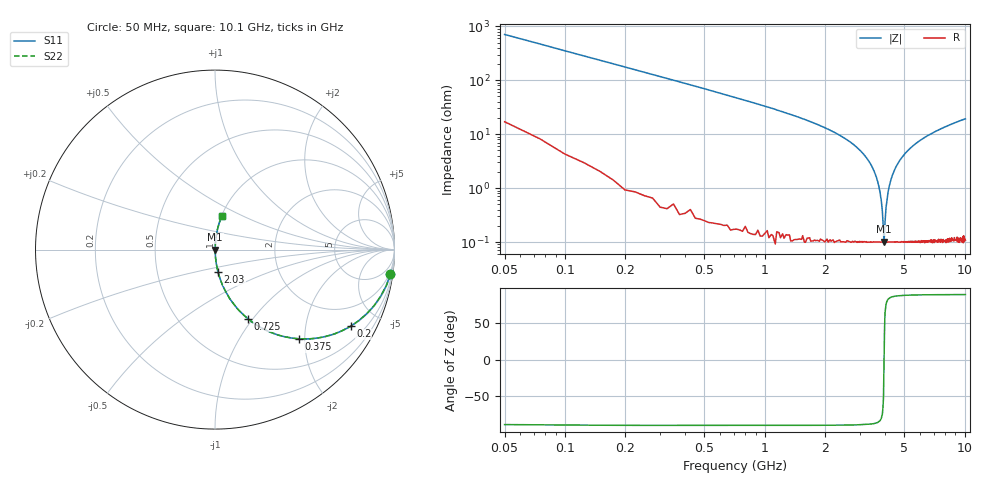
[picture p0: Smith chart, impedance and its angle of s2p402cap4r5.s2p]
! AVX Thin Film Operation		Date: April 2003
! Description: Accu-P® Series, Thin Film, SMD, RF Capacitor
! Part Number: 04025J4R5ABS
! 50 MHz  -  10.05 GHz
! Serial Measurements
# hz S db R 50
!	S11		S21		S12		S22
!	dB	Phase	dB	Phase	dB	Phase	dB	Phase
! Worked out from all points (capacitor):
!   400 points, 50 MHz to 10.1 GHz, reference 50 ohm
!   read as one part in series: C = 4.5 pF near 100 MHz
!   lowest |Z| = 102 mohm at 3.95 GHz (marker M1)
!   series resonance near 3.955 GHz, so ESL is about 360 pH
!   S11 on the Smith chart (normalised r, x): 50 MHz: 1, -14; 200 MHz: 1.02, -3.53; 375 MHz: 1.01, -1.87; 725 MHz: 1.00, -0.94; 2.03 GHz: 1.00, -0.26; 10.1 GHz: 1.00, +0.38
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5e7  -0.11 -8.0  -17.10 80.6  -17.10 80.6  -0.11 -8.0
1e8  -0.36 -15.7  -11.30 73.6  -11.30 73.6  -0.36 -15.7
2e8  -1.23 -29.5  -6.16 60.2  -6.16 60.2  -1.23 -29.5
3.75e8  -3.33 -46.8  -2.74 43.0  -2.74 43.0  -3.33 -46.8
7.25e8  -7.42 -64.6  -0.88 25.2  -0.88 25.2  -7.42 -64.6
1.73e9  -15.70 -80.2  -0.13 9.4  -0.13 9.4  -15.70 -80.2
2.03e9  -17.90 -82.2  -0.08 7.3  -0.08 7.3  -17.90 -82.2
2.78e9  -23.80 -85.4  -0.03 3.7  -0.03 3.7  -23.80 -85.4
3.4e9  -31.30 -86.3  -0.01 1.6  -0.01 1.6  -31.30 -86.3
3.63e9  -36.10 -85.4  -0.01 0.9  -0.01 0.9  -36.10 -85.4
3.78e9  -41.60 -82.7  -0.01 0.5  -0.01 0.5  -41.60 -82.7
3.88e9  -48.50 -74.4  -0.01 0.2  -0.01 0.2  -48.50 -74.4
3.95e9  -59.90 -10.8  -0.01 0.0  -0.01 0.0  -59.90 -10.8
3.98e9  -57.30 43.1  -0.01 -0.1  -0.01 -0.1  -57.30 43.1
4.05e9  -47.10 76.6  -0.01 -0.2  -0.01 -0.2  -47.10 76.6
4.15e9  -41.20 82.9  -0.01 -0.5  -0.01 -0.5  -41.20 82.9
4.25e9  -37.80 84.8  -0.01 -0.7  -0.01 -0.7  -37.80 84.8
4.6e9  -31.30 86.3  -0.01 -1.6  -0.01 -1.6  -31.30 86.3
5.08e9  -26.90 86.1  -0.02 -2.6  -0.02 -2.6  -26.90 86.1
6.75e9  -20.00 83.7  -0.05 -5.7  -0.05 -5.7  -20.00 83.7
8.43e9  -16.70 81.1  -0.10 -8.4  -0.10 -8.4  -16.70 81.1
1.01e10  -14.50 78.8  -0.17 -10.9  -0.17 -10.9  -14.50 78.8
